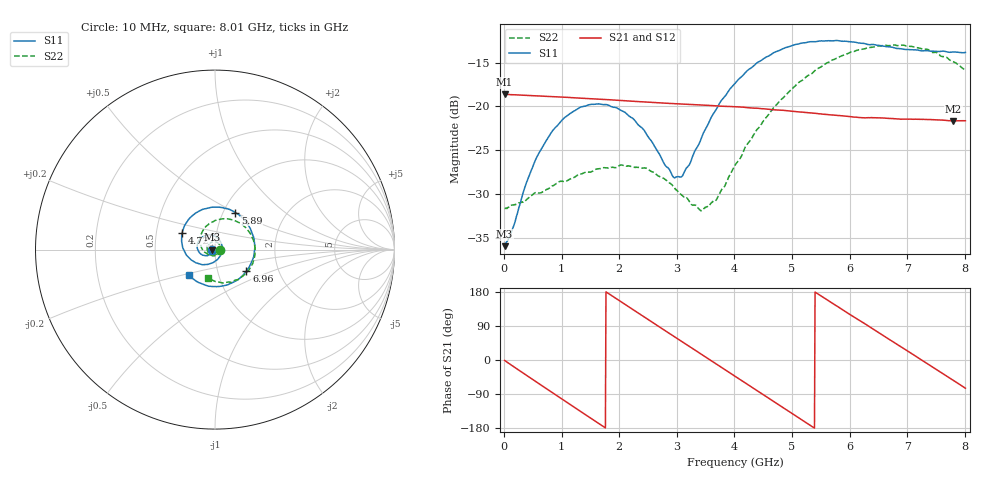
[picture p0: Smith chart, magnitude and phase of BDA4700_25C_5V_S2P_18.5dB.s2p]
!Agilent Technologies,E5071B,MY42404982,A.09.10
!Date: Mon Oct 20 13:35:35 2025
!Data & Calibration Information:
!Freq	S11:SOLT2(ON)	S21:SOLT2(ON)	S12:SOLT2(ON)	S22:SOLT2(ON)
# Hz S RI R 50
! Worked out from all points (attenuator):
!   801 points, 10 MHz to 8.01 GHz, reference 50 ohm
!   highest |S21| = -18.59 dB at 10 MHz (marker M1); lowest = -21.7 dB at 7.8 GHz (marker M2)
!   lowest |S11| = -36.0 dB at 10 MHz (marker M3), VSWR 1.03, Z = 48.4 - j0.118 ohm
!   |S11| at or under -10 dB: start of sweep to end of sweep
!   |S22| runs from -31.9 to -13.0 dB; largest |S21 - S12| = 0.00095
!   S11 on the Smith chart (normalised r, x): 10 MHz: 0.97, -0.00; 4.72 GHz: 0.68, +0.13; 5.89 GHz: 1.14, +0.50; 6.96 GHz: 1.38, -0.34; 8.01 GHz: 0.72, -0.21
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1e7  -0.0159 -0.00122  0.1176 -0.00256  0.1176 -0.00264  0.0261 -0.000874
1.4e8  -0.0172 -0.00948  0.1129 -0.0297  0.1128 -0.0298  0.0264 -0.00687
3.8e8  -0.0261 -0.0248  0.0895 -0.0734  0.0894 -0.0735  0.0212 -0.0199
6.2e8  -0.0435 -0.034  0.0506 -0.103  0.0505 -0.103  0.0112 -0.03
1.01e9  -0.0805 -0.0234  -0.0263 -0.1099  -0.0264 -0.1099  -0.0165 -0.0336
1.35e9  -0.0992 0.01  -0.0826 -0.0748  -0.0827 -0.0749  -0.0377 -0.0168
2.08e9  -0.0458 0.0815  -0.0923 0.056  -0.0923 0.0561  -0.0279 0.0364
2.68e9  0.0297 0.0456  0.00178 0.105  0.00174 0.1051  0.0169 0.0363
2.94e9  0.0391 0.00585  0.0467 0.0928  0.0467 0.0926  0.028 0.0209
3.08e9  0.0357 -0.0172  0.0673 0.0784  0.0669 0.0785  0.0299 0.00931
3.46e9  -0.00635 -0.0701  0.0997 0.0208  0.0997 0.0208  0.0165 -0.02
3.69e9  -0.0501 -0.0831  0.0989 -0.019  0.0989 -0.0193  -0.00229 -0.0293
4.01e9  -0.1174 -0.0673  0.0732 -0.0676  0.0733 -0.0675  -0.0367 -0.0276
4.72e9  -0.1838 0.0916  -0.038 -0.0877  -0.0377 -0.0879  -0.0835 0.058
5.35e9  -0.0599 0.2266  -0.0915 -0.00673  -0.0915 -0.00699  -0.0133 0.154
5.89e9  0.1137 0.2065  -0.0584 0.0663  -0.0584 0.0662  0.1125 0.1606
6.26e9  0.1977 0.1147  -0.00922 0.0856  -0.00837 0.0856  0.1888 0.0997
6.68e9  0.217 -0.0306  0.0489 0.0701  0.0491 0.0701  0.2226 -0.00882
6.96e9  0.1754 -0.1189  0.0746 0.0402  0.0747 0.0398  0.2063 -0.0845
7.37e9  0.0572 -0.1998  0.0824 -0.0172  0.0824 -0.0173  0.1288 -0.1669
7.8e9  -0.0911 -0.1834  0.0489 -0.0667  0.0488 -0.0669  0.0101 -0.1798
8.01e9  -0.1472 -0.1404  0.0221 -0.0799  0.0222 -0.0798  -0.0389 -0.1555
